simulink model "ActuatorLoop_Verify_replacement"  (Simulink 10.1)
settings: Solver=FixedStepDiscrete  StartTime=0.0  StopTime=10.0  RelTol=1e-3
undefined symbols (not defined in the file or in its folder): DiscIntNeverNeededParam, Kd, Ki, Kp, sldvsubsys, Ts
libraries: simulink x5, sldvlib x1

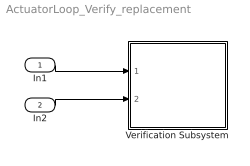
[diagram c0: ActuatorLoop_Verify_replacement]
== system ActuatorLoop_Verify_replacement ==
  In1 : Inport
  In2 : Inport  Port=2
  Verification Subsystem : Subsystem  Tag=VerificationSubsystem  DisableCoverage=on  LoadFcn=sldvsubsys('check')  TreatAsAtomicUnit=on  SimViewingDevice=on
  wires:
  In1/1 -> Verification Subsystem/1(In1)
  In2/1 -> Verification Subsystem/2(In2)

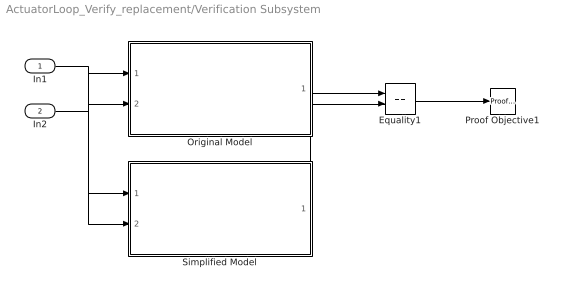
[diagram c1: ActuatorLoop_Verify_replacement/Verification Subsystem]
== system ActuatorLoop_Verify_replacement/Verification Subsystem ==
  In1 : Inport
  In2 : Inport  Port=2
  Equality1 : RelationalOperator  Operator===  OutDataTypeStr=boolean  RndMeth=Simplest
  Original Model : Subsystem  TreatAsAtomicUnit=on
  Proof Objective1 : sldvlib/Objectives and Constraints/Proof Objective  enabled=on  customAVTBlockType=Proof Objective  intervals=true  dispValues=on  outEnabled=off  enableStopSim=off
  Simplified Model : Subsystem  TreatAsAtomicUnit=on
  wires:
  In1/1 -> Original Model/1(pos), Simplified Model/1(pos)
  In2/1 -> Original Model/2(pos_cmd), Simplified Model/2(pos_cmd)
  Original Model/1(act_cmd) -> Equality1/1
  Simplified Model/1(act_cmd) -> Equality1/2
  Equality1/1 -> Proof Objective1/1

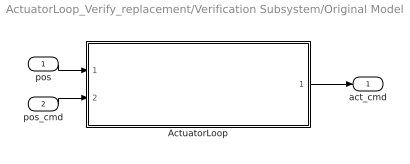
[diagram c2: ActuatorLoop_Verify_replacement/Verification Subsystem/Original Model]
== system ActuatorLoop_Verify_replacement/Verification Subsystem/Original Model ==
  pos : Inport  OutDataTypeStr=int16  PortDimensions=1  SampleTime=[0.001,0]
  pos_cmd : Inport  Port=2  OutDataTypeStr=double  PortDimensions=1  SampleTime=[0.001,0]
  ActuatorLoop : Subsystem  TreatAsAtomicUnit=on
  act_cmd : Outport  OutDataTypeStr=int16  PortDimensions=1  SampleTime=[0.001,0]
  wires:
  ActuatorLoop/1(ActuatorCommand) -> act_cmd/1
  pos_cmd/1 -> ActuatorLoop/2(PositionCommand)
  pos/1 -> ActuatorLoop/1(PositionFeedback)

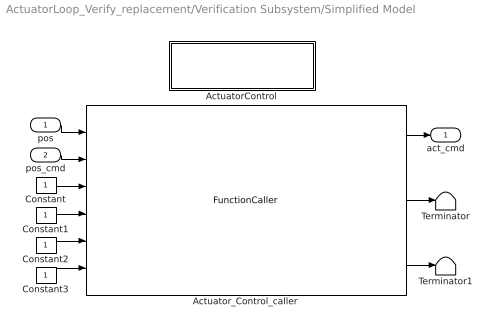
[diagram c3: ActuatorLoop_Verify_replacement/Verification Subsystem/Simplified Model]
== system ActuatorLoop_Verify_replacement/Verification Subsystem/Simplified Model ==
  pos : Inport  OutDataTypeStr=int16  PortDimensions=1  SampleTime=[0.001,0]
  pos_cmd : Inport  Port=2  OutDataTypeStr=double  PortDimensions=1  SampleTime=[0.001,0]
  ActuatorControl : Subsystem
  Actuator_Control_caller : FunctionCaller  FunctionPrototype=[Actuator1,Actuator2,Actuator3] = ActuatorControl.Actuator_Control(Act1_pos,Act1_cmd,Act2_pos,Act2_cmd,Act3_pos,Act3_cmd)  InputArgumentSpecifications=int16(1), double(1), int16(1), double(1), int16(1), double(1)  OutputArgumentSpecifications=int16(1), int16(1), int16(1)
  Constant : Constant  OutDataTypeStr=int16
  Constant1 : Constant  OutDataTypeStr=double
  Constant2 : Constant  OutDataTypeStr=int16
  Constant3 : Constant  OutDataTypeStr=double
  Terminator : Terminator
  Terminator1 : Terminator
  act_cmd : Outport  OutDataTypeStr=int16  PortDimensions=1  SampleTime=[0.001,0]
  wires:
  Actuator_Control_caller/1 -> act_cmd/1
  pos_cmd/1 -> Actuator_Control_caller/2
  pos/1 -> Actuator_Control_caller/1
  Constant3/1 -> Actuator_Control_caller/6
  Constant2/1 -> Actuator_Control_caller/5
  Constant1/1 -> Actuator_Control_caller/4
  Actuator_Control_caller/3 -> Terminator1/1
  Actuator_Control_caller/2 -> Terminator/1
  Constant/1 -> Actuator_Control_caller/3

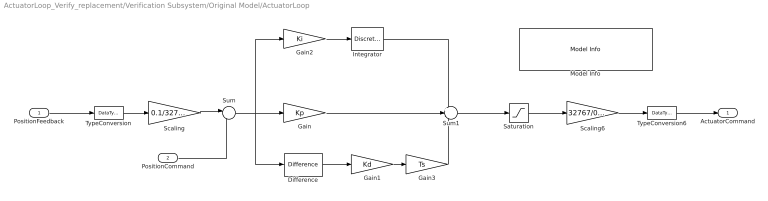
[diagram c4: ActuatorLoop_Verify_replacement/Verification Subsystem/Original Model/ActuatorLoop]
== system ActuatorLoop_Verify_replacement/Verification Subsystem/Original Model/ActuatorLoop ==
  PositionFeedback : Inport  OutMin=-32768  OutMax=32767  OutDataTypeStr=int16  PortDimensions=1  SampleTime=[0.001,0]
  PositionCommand : Inport  Port=2  OutMin=-0.1  OutMax=0.1  OutDataTypeStr=double  PortDimensions=1  SampleTime=[0.001,0]
  Difference : simulink/Discrete/Difference  ICPrevInput=0.0  OutMin=[]  OutMax=[]  OutDataType=fixdt(1, 16)  OutScaling=2^-10  DoSatur=off
  Gain : Gain  Gain=Kp
  Gain1 : Gain  Gain=Kd
  Gain2 : Gain  Gain=Ki
  Gain3 : Gain  Gain=Ts
  Integrator : DiscreteIntegrator  SampleTime=-1  LimitOutput=on  UpperSaturationLimit=0.1  LowerSaturationLimit=-0.1  ICPrevOutput=DiscIntNeverNeededParam  ICPrevScaledInput=DiscIntNeverNeededParam
  Model Info : simulink/Model-Wide Utilities/Model Info  Frame=on  DisplayStringWithTags=|  HorizontalTextAlignment=Center  LeftAlignmentValue=0.5
      | Model Name: %<ModelName>
      | Model Version: %<ModelVersion>
      | Last Modified: %<LastModificationDate>
      | 
      | Copyright 2016 The MathWorks, Inc.
  Saturation : Saturate  UpperLimit=0.3  LowerLimit=-0.3
  Scaling : Gain  Gain=0.1/32767
  Scaling6 : Gain  Gain=32767/0.3  SaturateOnIntegerOverflow=on
  Sum : Sum  Inputs=|-+
  Sum1 : Sum  Inputs=++-
  TypeConversion : DataTypeConversion  OutDataTypeStr=double
  TypeConversion6 : DataTypeConversion  OutDataTypeStr=int16
  ActuatorCommand : Outport  OutDataTypeStr=int16  PortDimensions=1  SampleTime=[0.001,0]  VectorParamsAs1DForOutWhenUnconnected=off
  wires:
  Gain3/1 -> Sum1/3
  TypeConversion6/1 -> ActuatorCommand/1
  Saturation/1 -> Scaling6/1
  Scaling6/1 -> TypeConversion6/1
  Scaling/1 -> Sum/1
  TypeConversion/1 -> Scaling/1
  PositionFeedback/1 -> TypeConversion/1
  Gain2/1 -> Integrator/1
  Gain1/1 -> Gain3/1
  Difference/1 -> Gain1/1
  Integrator/1 -> Sum1/1
  Sum1/1 -> Saturation/1
  Gain/1 -> Sum1/2
  Sum/1 -> Difference/1, Gain2/1, Gain/1
  PositionCommand/1 -> Sum/2

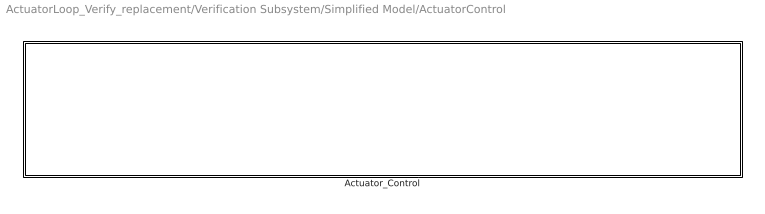
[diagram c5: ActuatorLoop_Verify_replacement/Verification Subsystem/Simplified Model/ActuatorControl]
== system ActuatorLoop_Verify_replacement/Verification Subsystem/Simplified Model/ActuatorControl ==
  Actuator_Control : Subsystem  TreatAsAtomicUnit=on

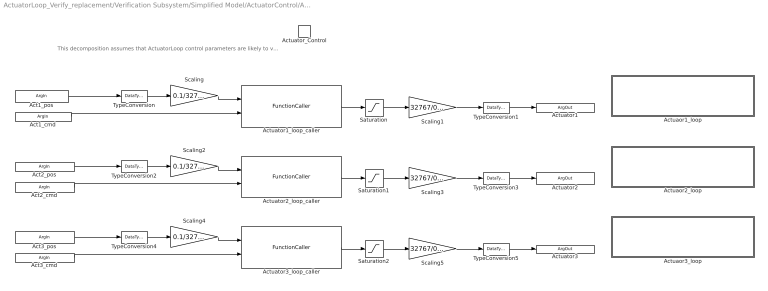
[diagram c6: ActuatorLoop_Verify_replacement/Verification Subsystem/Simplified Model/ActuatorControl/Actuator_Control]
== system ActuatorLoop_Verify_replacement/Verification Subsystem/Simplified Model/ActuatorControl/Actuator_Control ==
  note: This decomposition assumes that ActuatorLoop control parameters are likely to vary between actuators.
  Actuator_Control : TriggerPort  TriggerType=function-call  IsSimulinkFunction=on  FunctionName=Actuator_Control  FunctionVisibility=scoped  VariantControl=Variant  PortDimensions=1
  Actuaor1_loop : Subsystem  TreatAsAtomicUnit=on
  Actuaor2_loop : Subsystem  TreatAsAtomicUnit=on
  Actuaor3_loop : Subsystem  TreatAsAtomicUnit=on
  Actuator1_loop_caller : FunctionCaller  FunctionPrototype=Actuator1 = Actuator1_loop(Act1_pos,Act1_cmd)  InputArgumentSpecifications=double(1), double(1)  OutputArgumentSpecifications=double(1)
  Actuator2_loop_caller : FunctionCaller  FunctionPrototype=Actuator2 = Actuator2_loop(Act2_pos,Act2_cmd)  InputArgumentSpecifications=double(1), double(1)  OutputArgumentSpecifications=double(1)
  Actuator3_loop_caller : FunctionCaller  FunctionPrototype=Actuator3 = Actuator3_loop(Act3_pos,Act3_cmd)  InputArgumentSpecifications=double(1), double(1)  OutputArgumentSpecifications=double(1)
  Saturation : Saturate  UpperLimit=0.3  LowerLimit=-0.3
  Saturation1 : Saturate  UpperLimit=0.3  LowerLimit=-0.3
  Saturation2 : Saturate  UpperLimit=0.3  LowerLimit=-0.3
  Scaling : Gain  Gain=0.1/32767
  Scaling1 : Gain  Gain=32767/0.3  SaturateOnIntegerOverflow=on
  Scaling2 : Gain  Gain=0.1/32767
  Scaling3 : Gain  Gain=32767/0.3  SaturateOnIntegerOverflow=on
  Scaling4 : Gain  Gain=0.1/32767
  Scaling5 : Gain  Gain=32767/0.3  SaturateOnIntegerOverflow=on
  TypeConversion : DataTypeConversion  OutDataTypeStr=double
  TypeConversion1 : DataTypeConversion  OutDataTypeStr=int16
  TypeConversion2 : DataTypeConversion  OutDataTypeStr=double
  TypeConversion3 : DataTypeConversion  OutDataTypeStr=int16
  TypeConversion4 : DataTypeConversion  OutDataTypeStr=double
  TypeConversion5 : DataTypeConversion  OutDataTypeStr=int16
  Act1_pos : ArgIn  OutDataTypeStr=int16  ArgumentName=Act1_pos
  Act1_cmd : ArgIn  Port=2  ArgumentName=Act1_cmd
  Act2_pos : ArgIn  Port=3  OutDataTypeStr=int16  ArgumentName=Act2_pos
  Act2_cmd : ArgIn  Port=4  ArgumentName=Act2_cmd
  Act3_pos : ArgIn  Port=5  OutDataTypeStr=int16  ArgumentName=Act3_pos
  Act3_cmd : ArgIn  Port=6  ArgumentName=Act3_cmd
  Actuator1 : ArgOut  OutMin=-32768  OutMax=32767  OutDataTypeStr=int16  ArgumentName=Actuator1
  Actuator2 : ArgOut  Port=2  OutMin=-32768  OutMax=32767  OutDataTypeStr=int16  ArgumentName=Actuator2
  Actuator3 : ArgOut  Port=3  OutMin=-32768  OutMax=32767  OutDataTypeStr=int16  ArgumentName=Actuator3
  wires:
  Actuator1_loop_caller/1 -> Saturation/1
  Saturation/1 -> Scaling1/1
  Scaling/1 -> Actuator1_loop_caller/1
  Scaling1/1 -> TypeConversion1/1
  Act1_pos/1 -> TypeConversion/1
  TypeConversion1/1 -> Actuator1/1
  TypeConversion/1 -> Scaling/1
  Scaling3/1 -> TypeConversion3/1
  TypeConversion2/1 -> Scaling2/1
  TypeConversion3/1 -> Actuator2/1
  Scaling2/1 -> Actuator2_loop_caller/1
  Saturation1/1 -> Scaling3/1
  Act2_pos/1 -> TypeConversion2/1
  Actuator2_loop_caller/1 -> Saturation1/1
  Actuator3_loop_caller/1 -> Saturation2/1
  Scaling5/1 -> TypeConversion5/1
  Saturation2/1 -> Scaling5/1
  Act3_pos/1 -> TypeConversion4/1
  Scaling4/1 -> Actuator3_loop_caller/1
  TypeConversion5/1 -> Actuator3/1
  TypeConversion4/1 -> Scaling4/1
  Act1_cmd/1 -> Actuator1_loop_caller/2
  Act2_cmd/1 -> Actuator2_loop_caller/2
  Act3_cmd/1 -> Actuator3_loop_caller/2

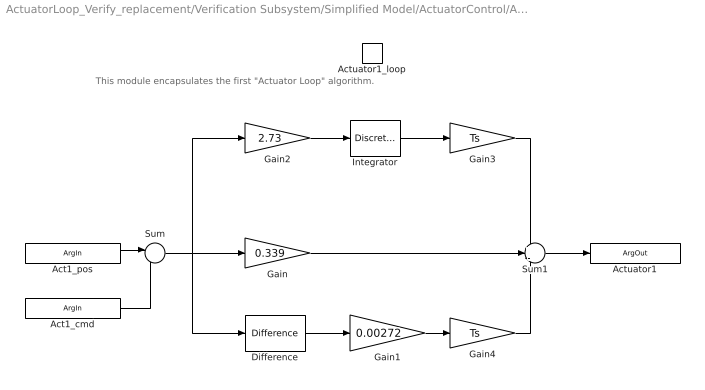
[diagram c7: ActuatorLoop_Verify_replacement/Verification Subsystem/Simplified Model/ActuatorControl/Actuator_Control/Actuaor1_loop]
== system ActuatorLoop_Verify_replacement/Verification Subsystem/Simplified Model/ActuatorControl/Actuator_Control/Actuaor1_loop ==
  note: This module encapsulates the first "Actuator Loop" algorithm.
  Actuator1_loop : TriggerPort  TriggerType=function-call  IsSimulinkFunction=on  FunctionName=Actuator1_loop  FunctionVisibility=scoped  VariantControl=Variant  PortDimensions=1
  Difference : simulink/Discrete/Difference  ICPrevInput=0.0  OutMin=[]  OutMax=[]  OutDataType=fixdt(1, 16)  OutScaling=2^-10  DoSatur=off
  Gain : Gain  Gain=0.339
  Gain1 : Gain  Gain=0.00272
  Gain2 : Gain  Gain=2.73
  Gain3 : Gain  Gain=Ts
  Gain4 : Gain  Gain=Ts
  Integrator : DiscreteIntegrator  IntegratorMethod=Accumulation: Forward Euler  SampleTime=-1  LimitOutput=on  UpperSaturationLimit=0.1  LowerSaturationLimit=-0.1  ICPrevOutput=DiscIntNeverNeededParam  ICPrevScaledInput=DiscIntNeverNeededParam
  Sum : Sum  Inputs=|-+
  Sum1 : Sum  Inputs=++-
  Act1_pos : ArgIn  ArgumentName=Act1_pos
  Act1_cmd : ArgIn  Port=2  ArgumentName=Act1_cmd
  Actuator1 : ArgOut  ArgumentName=Actuator1
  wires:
  Gain1/1 -> Gain4/1
  Sum1/1 -> Actuator1/1
  Integrator/1 -> Gain3/1
  Gain2/1 -> Integrator/1
  Gain/1 -> Sum1/2
  Difference/1 -> Gain1/1
  Gain3/1 -> Sum1/1
  Gain4/1 -> Sum1/3
  Act1_pos/1 -> Sum/1
  Sum/1 -> Difference/1, Gain2/1, Gain/1
  Act1_cmd/1 -> Sum/2

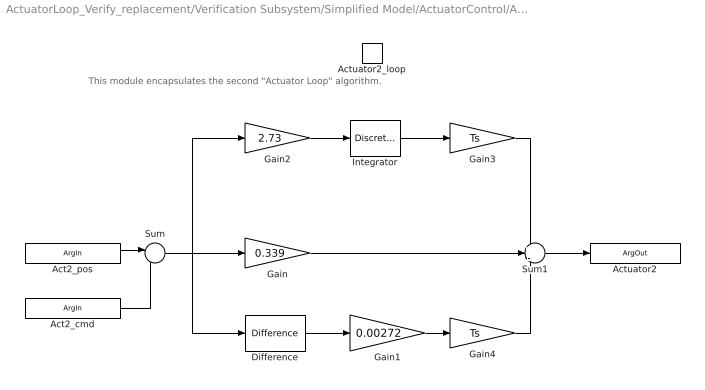
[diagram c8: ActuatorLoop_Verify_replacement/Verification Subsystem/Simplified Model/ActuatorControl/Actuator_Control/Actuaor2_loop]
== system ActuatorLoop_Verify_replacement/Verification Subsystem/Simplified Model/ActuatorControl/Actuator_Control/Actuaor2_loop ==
  note: This module encapsulates the second "Actuator Loop" algorithm.
  Actuator2_loop : TriggerPort  TriggerType=function-call  IsSimulinkFunction=on  FunctionName=Actuator2_loop  FunctionVisibility=scoped  VariantControl=Variant  PortDimensions=1
  Difference : simulink/Discrete/Difference  ICPrevInput=0.0  OutMin=[]  OutMax=[]  OutDataType=fixdt(1, 16)  OutScaling=2^-10  DoSatur=off
  Gain : Gain  Gain=0.339
  Gain1 : Gain  Gain=0.00272
  Gain2 : Gain  Gain=2.73
  Gain3 : Gain  Gain=Ts
  Gain4 : Gain  Gain=Ts
  Integrator : DiscreteIntegrator  IntegratorMethod=Accumulation: Forward Euler  SampleTime=-1  LimitOutput=on  UpperSaturationLimit=0.1  LowerSaturationLimit=-0.1  ICPrevOutput=DiscIntNeverNeededParam  ICPrevScaledInput=DiscIntNeverNeededParam
  Sum : Sum  Inputs=|-+
  Sum1 : Sum  Inputs=++-
  Act2_pos : ArgIn  ArgumentName=Act2_pos
  Act2_cmd : ArgIn  Port=2  ArgumentName=Act2_cmd
  Actuator2 : ArgOut  ArgumentName=Actuator2
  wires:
  Act2_cmd/1 -> Sum/2
  Sum/1 -> Gain/1, Gain2/1, Difference/1
  Act2_pos/1 -> Sum/1
  Gain4/1 -> Sum1/3
  Gain3/1 -> Sum1/1
  Difference/1 -> Gain1/1
  Gain/1 -> Sum1/2
  Gain2/1 -> Integrator/1
  Integrator/1 -> Gain3/1
  Sum1/1 -> Actuator2/1
  Gain1/1 -> Gain4/1

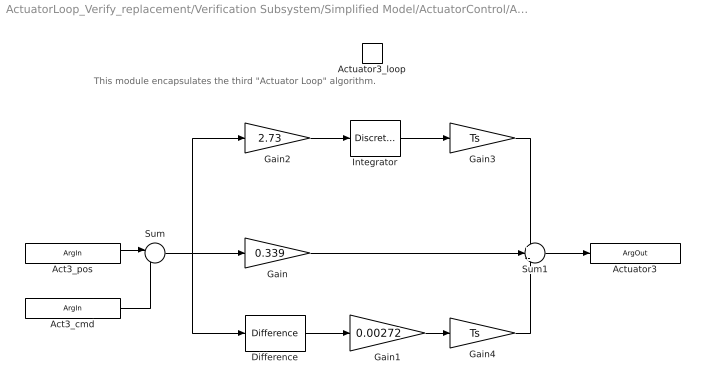
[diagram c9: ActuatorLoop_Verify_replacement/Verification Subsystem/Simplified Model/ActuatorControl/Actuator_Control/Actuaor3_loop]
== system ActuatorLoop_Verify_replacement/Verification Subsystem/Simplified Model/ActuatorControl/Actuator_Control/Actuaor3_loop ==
  note: This module encapsulates the third "Actuator Loop" algorithm.
  Actuator3_loop : TriggerPort  TriggerType=function-call  IsSimulinkFunction=on  FunctionName=Actuator3_loop  FunctionVisibility=scoped  VariantControl=Variant  PortDimensions=1
  Difference : simulink/Discrete/Difference  ICPrevInput=0.0  OutMin=[]  OutMax=[]  OutDataType=fixdt(1, 16)  OutScaling=2^-10  DoSatur=off
  Gain : Gain  Gain=0.339
  Gain1 : Gain  Gain=0.00272
  Gain2 : Gain  Gain=2.73
  Gain3 : Gain  Gain=Ts
  Gain4 : Gain  Gain=Ts
  Integrator : DiscreteIntegrator  IntegratorMethod=Accumulation: Forward Euler  SampleTime=-1  LimitOutput=on  UpperSaturationLimit=0.1  LowerSaturationLimit=-0.1  ICPrevOutput=DiscIntNeverNeededParam  ICPrevScaledInput=DiscIntNeverNeededParam
  Sum : Sum  Inputs=|-+
  Sum1 : Sum  Inputs=++-
  Act3_pos : ArgIn  ArgumentName=Act3_pos
  Act3_cmd : ArgIn  Port=2  ArgumentName=Act3_cmd
  Actuator3 : ArgOut  ArgumentName=Actuator3
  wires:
  Gain1/1 -> Gain4/1
  Sum1/1 -> Actuator3/1
  Integrator/1 -> Gain3/1
  Gain2/1 -> Integrator/1
  Gain/1 -> Sum1/2
  Difference/1 -> Gain1/1
  Gain3/1 -> Sum1/1
  Gain4/1 -> Sum1/3
  Act3_pos/1 -> Sum/1
  Sum/1 -> Difference/1, Gain2/1, Gain/1
  Act3_cmd/1 -> Sum/2
